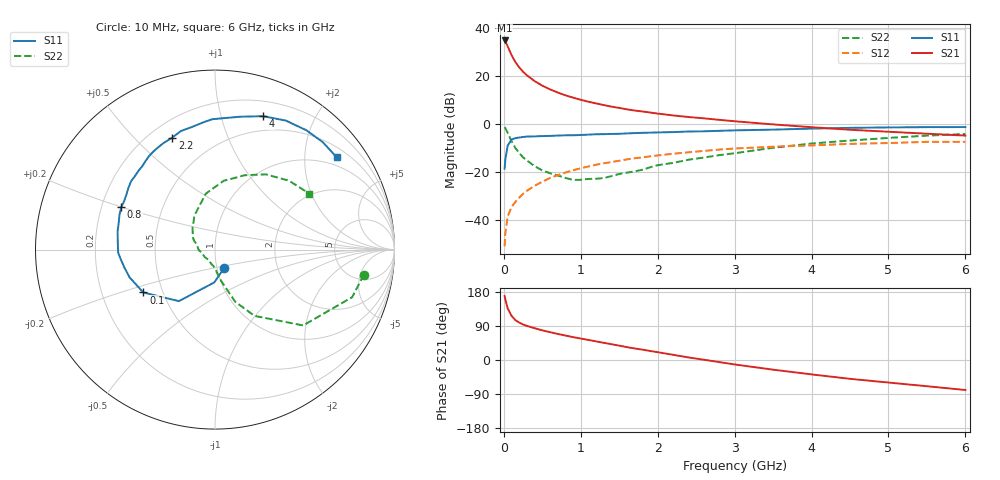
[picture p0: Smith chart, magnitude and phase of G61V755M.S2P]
! SIEMENS Small Signal Semiconductors
! BFG193
! Si NPN RF Bipolar Junction Transistor in SOT223
! VCE = 1.75 V  IC = 55 mA
! Common Emitter S-Parameters:  August  1996
# GHz  S  MA  R  50
!  f  S11  S21  S12  S22
! GHz  MAG  ANG  MAG  ANG  MAG  ANG  MAG  ANG
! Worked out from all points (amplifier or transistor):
!   36 points, 10 MHz to 6 GHz, reference 50 ohm
!   highest |S21| = 34.7 dB at 10 MHz (marker M1)
!   |S21| within 3 dB of that: start of sweep to 57.39 MHz
!   unconditionally stable (mu >= 1): 311.3 MHz to 2.705 GHz
!   at 250 MHz: K = 0.97, MSG = 25.4 dB, |S12| = -29.2 dB
!   at 1.4 GHz: K = 1.07, MAG = 9.9 dB, |S12| = -16.0 dB
!   at 6 GHz: K = 0.96, MSG = 1.3 dB, |S12| = -7.5 dB
!   S11 on the Smith chart (normalised r, x): 10 MHz: 1.08, -0.23; 100 MHz: 0.39, -0.24; 800 MHz: 0.28, +0.20; 2.2 GHz: 0.29, +0.65; 4 GHz: 0.35, +1.37; 6 GHz: 0.75, +2.79
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0.01  0.1158 -64.2  54.39 169.2  0.0028 87.8  0.8413 -9.5
0.02  0.1832 -91.4  51.85 159.6  0.0053 72.4  0.8091 -19.1
0.05  0.3506 -125.0  40.95 136.3  0.0116 66.3  0.6479 -40.7
0.1  0.4654 -149.1  27 116.5  0.0184 63.4  0.43 -59.2
0.15  0.5005 -162.0  19.22 105.1  0.0234 63.0  0.3121 -68.7
0.2  0.515 -169.0  14.95 98.8  0.0287 66.1  0.2456 -72.4
0.25  0.5292 -174.6  12.11 93.8  0.0347 66.6  0.198 -76.5
0.3  0.5399 -178.3  10.2 90.0  0.04 67.4  0.1715 -79.7
0.4  0.5442 174.9  7.735 83.9  0.0508 67.7  0.1306 -84.9
0.5  0.5523 169.1  6.209 78.3  0.0618 67.1  0.106 -89.3
0.6  0.5571 164.3  5.199 73.5  0.0739 66.1  0.0932 -94.9
0.7  0.5661 160.1  4.476 68.8  0.0844 64.7  0.0836 -103.3
0.8  0.5733 155.7  3.911 64.6  0.0959 62.6  0.0742 -112.9
1.1  0.5923 144.5  2.873 52.9  0.1283 57.0  0.0706 -142.2
1.6  0.6279 127.9  1.992 34.0  0.1802 45.6  0.0954 174.8
2.2  0.6682 110.9  1.487 13.7  0.2365 31.3  0.1524 144.5
2.8  0.7108 95.6  1.205 -5.5  0.2891 16.9  0.2215 121.3
3.5  0.7528 79.5  0.967 -25.5  0.3314 -1.0  0.3158 99.3
4  0.7901 70.2  0.846 -38.0  0.3526 -10.8  0.3862 82.8
4.5  0.8201 61.2  0.748 -49.7  0.3802 -21.0  0.4458 68.3
5.5  0.8479 45.0  0.619 -69.2  0.4188 -44.1  0.5638 42.9
6  0.8511 37.2  0.565 -79.2  0.4199 -57.3  0.6113 30.6
